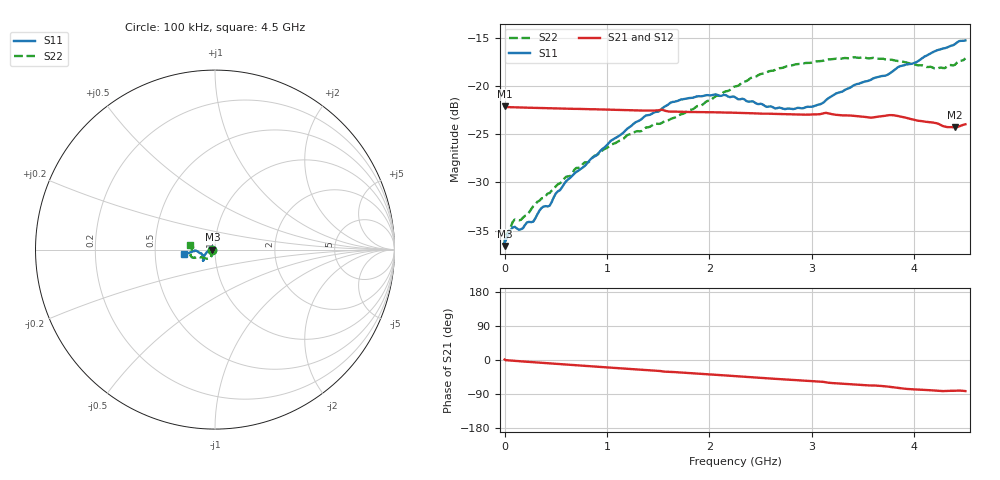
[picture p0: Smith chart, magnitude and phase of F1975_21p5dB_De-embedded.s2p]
! Integrated Device Technology
! Corporate Headquarters
! 6024 Silver Creek Valley Road
! San Jose, CA 95138  USA
! Phone:  1-408-284-8200
! Toll Free:  1-800-223-1366
! Webpage:  http://www.idt.com/
! Timing and RF Division
! 515 Groton Road, Suite 102
! Westford, MA 01886-6024
! Device:  F1975
! Description: 6-bit, 75 ohm, 0.5 dB Digital Step Attenuator
! Frequency:  5.0 MHz -  3.00 GHz
! Package:  4x4 mm QFN Plastic Package: 20 pin
! Ports:  2 RF, 11 DC
!  Pin  1  = D5 (16 dB)
!  Pin  2  = RF1  =  Port 1
!  Pin  3  = Serial Data In (DATA)
!  Pin  4  = Serial Clock (CLK)
!  Pin  5  = Serial Latch Enable (LE)
!  Pin  6  = VDD
!  Pin  7  = NC
!  Pin  8  = NC
!  Pin  9  = NC
!  Pin 10  = GND
!  Pin 11  = GND
!  Pin 12  = NC
!  Pin 13  = VMODE
!  Pin 14  = RF2  =  Port 2
!  Pin 15  = D4 (8 dB)
!  Pin 16  = D3 (4 dB)
!  Pin 17  = D2 (2 dB)
!  Pin 18  = NC
!  Pin 19  = D1 (1 dB)
!  Pin 20  = D0 (0.5 dB)
! State:  43
! Atten State:  21.5 dB
! Voltage:  +3.30 Volts
! Current:  0.566 mA
! Data:  The device was measured on a F1975 evaluation board which has
!  individual transmission lines to the RF pins.  Data was collected
!  using a calibrated network analyzer.  The evaluation board was
!  de-embedded using Automatic Fixture Removal (AFR).
!  The reference plane is the edge of the package pin.
! Misc:
!  Action Tracker AT0415
! Date Measured:  2018-02-08
! Date:  2018-03-26  MJV
! Note:
!  Integrated Device Technology supplies this data as a sample of measured
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# GHz S dB R 75
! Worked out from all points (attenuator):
!   291 points, 100 kHz to 4.5 GHz, reference 75 ohm
!   highest |S21| = -22.10 dB at 200 kHz (marker M1); lowest = -24.3 dB at 4.4 GHz (marker M2)
!   lowest |S11| = -36.6 dB at 100 kHz (marker M3), VSWR 1.03, Z = 72.8 - j0.0169 ohm
!   |S11| at or under -10 dB: start of sweep to end of sweep
!   |S22| runs from -36.6 to -17.0 dB; largest |S21 - S12| = 0.00014
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0.0001  -36.59 -179.6  -22.10 1.2  -22.11 1.2  -36.61 -178.5
0.0002  -36.48 -179.6  -22.10 1.2  -22.11 1.2  -36.54 -178.4
0.009  -35.99 -178.4  -22.17 -0.2  -22.17 -0.2  -35.60 -174.8
0.1  -34.60 -175.3  -22.21 -2.2  -22.20 -2.2  -33.84 -158.5
0.16  -34.85 -177.1  -22.23 -3.5  -22.23 -3.5  -33.87 -150.0
0.28  -34.06 179.8  -22.26 -5.8  -22.26 -5.8  -32.46 -139.7
0.36  -32.65 179.9  -22.28 -7.4  -22.28 -7.4  -31.66 -131.8
0.44  -32.41 -179.5  -22.30 -8.9  -22.30 -8.9  -31.09 -126.1
0.6  -29.89 -175.7  -22.35 -12.0  -22.34 -12.0  -29.41 -122.0
0.76  -28.48 -168.8  -22.38 -15.0  -22.38 -15.0  -28.14 -120.0
1.28  -23.75 -152.4  -22.52 -24.7  -22.52 -24.7  -24.71 -121.2
1.52  -22.53 -144.5  -22.48 -29.1  -22.47 -29.1  -23.92 -128.0
1.62  -21.73 -142.7  -22.66 -31.4  -22.65 -31.4  -23.43 -131.6
1.88  -21.07 -138.6  -22.70 -35.7  -22.70 -35.7  -22.08 -143.3
2.26  -21.22 -137.7  -22.77 -42.7  -22.76 -42.7  -20.02 -154.6
2.64  -22.32 -147.1  -22.89 -49.7  -22.88 -49.6  -18.34 -158.2
3.02  -22.09 -163.6  -22.94 -56.2  -22.94 -56.2  -17.52 -160.9
3.42  -19.87 -175.1  -23.11 -64.9  -23.11 -64.9  -17.02 -166.8
3.76  -18.70 -175.6  -23.02 -70.8  -23.02 -70.8  -17.27 -173.5
4.2  -16.40 -172.4  -23.82 -80.7  -23.82 -80.7  -18.19 174.5
4.4  -15.64 -170.4  -24.29 -81.1  -24.29 -81.1  -17.78 171.2
4.5  -15.27 -172.1  -23.97 -82.0  -23.96 -82.0  -17.13 169.7
